// ------------------------------------------------------------------
// File           : C:\Programmi\Siemens\NCVar Selector\GANTRY.awl
//
// Source File    : C:\Programmi\Siemens\NCVar Selector\GANTRY.var
// Generation Date: 20/09/2016  Time: 13.04.07
// ------------------------------------------------------------------

DATA_BLOCK DB  123
VERSION : 0.0


STRUCT

 A2_M_GANTRY_BREAK_UP:
   STRUCT
   SYNTAX_ID : BYTE  := B#16#82;
   bereich_u_einheit : BYTE := B#16#62;
   spalte : WORD := W#16#9114;
   zeile : WORD := W#16#1;
   bausteintyp : BYTE := B#16#1A;
   ZEILENANZAHL : BYTE := B#16#1;
   typ : BYTE := B#16#1;
   laenge : BYTE := B#16#1;
   END_STRUCT ;

 A3_M_GANTRY_BREAK_UP:
   STRUCT
   SYNTAX_ID : BYTE  := B#16#82;
   bereich_u_einheit : BYTE := B#16#63;
   spalte : WORD := W#16#9114;
   zeile : WORD := W#16#1;
   bausteintyp : BYTE := B#16#1A;
   ZEILENANZAHL : BYTE := B#16#1;
   typ : BYTE := B#16#1;
   laenge : BYTE := B#16#1;
   END_STRUCT ;

 END_STRUCT ;

BEGIN
END_DATA_BLOCK
